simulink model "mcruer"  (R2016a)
settings: Solver=ode5  StartTime=0.0  StopTime=60.0  FixedStep=0.001  RelTol=1e-3
undefined symbols (not defined in the file): initialv, initialy, K_cd, K_p, T_I, T_L, T_N, tau, tau2

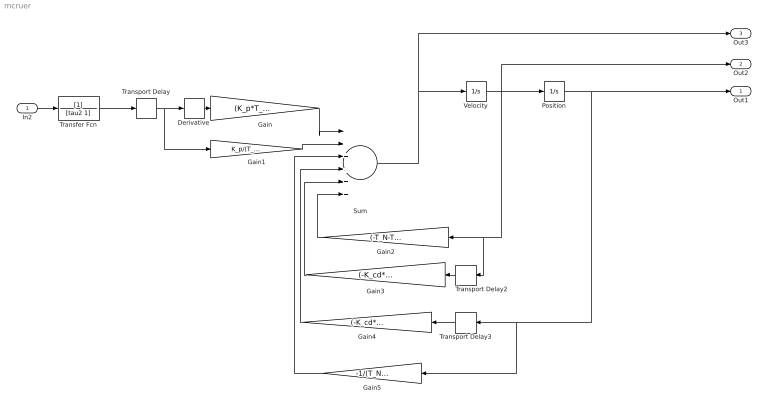
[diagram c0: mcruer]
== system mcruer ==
  In2 : Inport
  Derivative : Derivative
  Gain : Gain  Gain=(K_p*T_L)/(T_N*T_I)
  Gain1 : Gain  Gain=K_p/(T_N*T_I)
  Gain2 : Gain  Gain=(-T_N-T_I)/(T_N*T_I)
  Gain3 : Gain  Gain=(-K_cd*K_p*T_L)/(T_N*T_I)
  Gain4 : Gain  Gain=(-K_cd*K_p)/(T_N*T_I)
  Gain5 : Gain  Gain=-1/(T_N*T_I)
  Position : Integrator  InitialCondition=initialy
  Sum : Sum  Inputs=|++++++
  Transfer Fcn : TransferFcn  Denominator=[tau2 1]
  Transport Delay : TransportDelay  DelayTime=tau
  Transport Delay2 : TransportDelay  DelayTime=tau
  Transport Delay3 : TransportDelay  DelayTime=tau
  Velocity : Integrator  InitialCondition=initialv
  Out1 : Outport
  Out2 : Outport  Port=2
  Out3 : Outport  Port=3
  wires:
  In2/1 -> Transfer Fcn/1
  Velocity/1 -> Out2/1, Position/1, Gain2/1, Transport Delay2/1
  Transport Delay/1 -> Gain1/1, Derivative/1
  Derivative/1 -> Gain/1
  Gain/1 -> Sum/1
  Gain1/1 -> Sum/2
  Gain2/1 -> Sum/6
  Transport Delay2/1 -> Gain3/1
  Gain3/1 -> Sum/5
  Transport Delay3/1 -> Gain4/1
  Gain4/1 -> Sum/4
  Gain5/1 -> Sum/3
  Sum/1 -> Out3/1, Velocity/1
  Position/1 -> Out1/1, Gain5/1, Transport Delay3/1
  Transfer Fcn/1 -> Transport Delay/1
